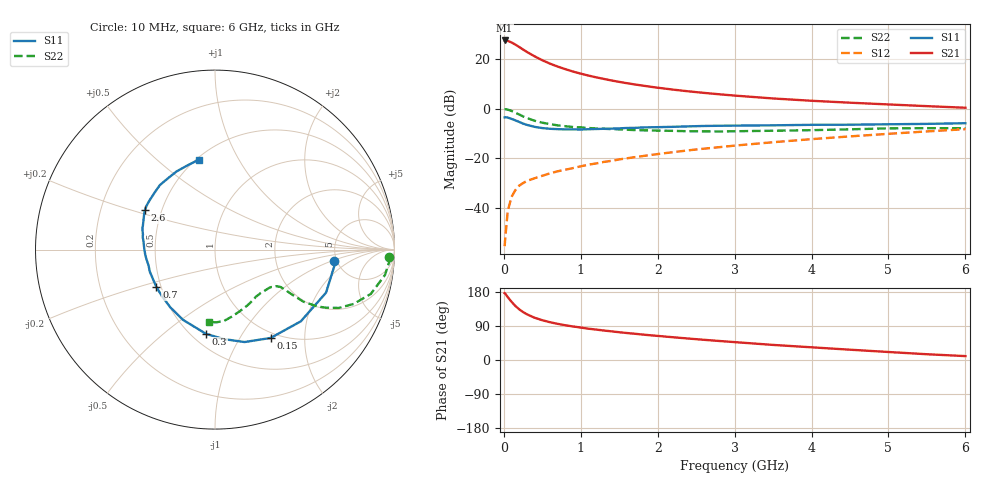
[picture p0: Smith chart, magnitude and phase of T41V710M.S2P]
! Infineon Technologies  Discrete & RF Semiconductors
! BFR182T
! Si NPN RF Bipolar Junction Transistor in SC75
! VCE = 1.75 V  IC = 10 mA
! Common Emitter S-Parameters:  October  1999
# GHz  S  MA  R  50
!  f  S11  S21  S12  S22
! GHz  MAG  ANG  MAG  ANG  MAG  ANG  MAG  ANG
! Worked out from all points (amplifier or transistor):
!   36 points, 10 MHz to 6 GHz, reference 50 ohm
!   highest |S21| = 27.5 dB at 10 MHz (marker M1)
!   |S21| within 3 dB of that: start of sweep to 218.1 MHz
!   unconditionally stable (mu >= 1): 894.2 MHz to 3.816 GHz
!   at 250 MHz: K = 0.47, MSG = 26.9 dB, |S12| = -30.0 dB
!   at 1.4 GHz: K = 1.10, MAG = 14.3 dB, |S12| = -21.0 dB
!   at 6 GHz: K = 0.85, MSG = 4.3 dB, |S12| = -8.3 dB
!   lowest NFmin = 1.50 dB at 450 MHz
!   S11 on the Smith chart (normalised r, x): 10 MHz: 4.76, -1.08; 150 MHz: 0.92, -1.37; 300 MHz: 0.59, -0.71; 700 MHz: 0.47, -0.23; 2.6 GHz: 0.40, +0.22; 6 GHz: 0.52, +0.70
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0.01  0.6674 -5.4  23.67 176.3  0.0017 76.5  0.9712 -2.4
0.02  0.6723 -7.2  23.5 174.6  0.0026 89.3  0.9759 -3.4
0.05  0.6635 -21.2  23.21 166.0  0.0086 84.8  0.9576 -8.5
0.1  0.6231 -39.9  21.58 153.6  0.0167 74.1  0.9023 -15.9
0.15  0.5817 -57.8  19.54 142.5  0.0229 66.9  0.8296 -21.4
0.2  0.5407 -72.3  17.49 133.7  0.0282 65.1  0.763 -25.2
0.25  0.4999 -84.8  15.55 126.5  0.0317 59.8  0.6992 -27.6
0.3  0.472 -96.1  13.91 120.6  0.035 59.1  0.6502 -29.1
0.4  0.43 -114.5  11.34 111.5  0.0397 57.1  0.5713 -30.5
0.5  0.4068 -127.7  9.465 105.0  0.0445 57.6  0.5226 -30.3
0.6  0.3935 -138.6  8.074 99.7  0.0498 58.1  0.4878 -30.2
0.7  0.3871 -147.6  7.051 95.4  0.0548 59.9  0.4615 -29.9
0.9  0.3834 -161.5  5.592 88.5  0.0636 61.8  0.4274 -29.7
1.1  0.3857 -172.1  4.643 82.6  0.0745 63.1  0.4082 -30.3
1.3  0.3935 179.8  3.975 77.8  0.0846 64.2  0.3928 -31.5
1.6  0.4088 170.2  3.26 71.2  0.1001 65.3  0.3763 -33.7
2.2  0.4312 157.4  2.422 60.0  0.1331 66.3  0.3572 -40.8
2.6  0.4485 150.4  2.081 53.3  0.1563 66.0  0.3494 -46.2
3.5  0.4622 137.0  1.606 39.8  0.211 63.4  0.3594 -59.6
4.5  0.4754 124.0  1.32 27.2  0.2766 58.9  0.384 -75.4
5.5  0.4942 107.8  1.125 15.2  0.3485 53.0  0.4053 -89.1
6  0.5095 99.9  1.044 10.3  0.3866 49.1  0.4039 -94.7
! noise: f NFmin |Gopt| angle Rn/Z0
0.45  1.5  0.26  43  0.28
0.9  1.6  0.24  87  0.22
1.8  2.1  0.2  170  0.2
